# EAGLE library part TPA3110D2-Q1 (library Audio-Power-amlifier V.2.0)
15-W Filter-Free Stereo Class-D Audio Power Amplifier with SpeakerGuard
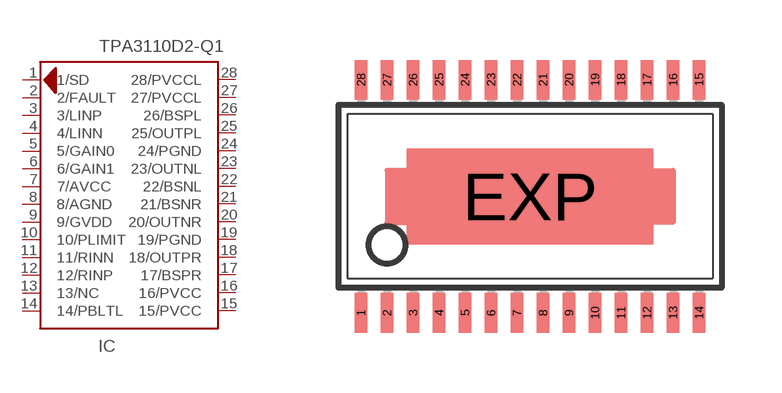
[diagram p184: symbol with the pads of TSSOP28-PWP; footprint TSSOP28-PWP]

Designator prefix IC

## TPA3110D2-Q1  [TSSOP28-PWP]
1  1/SD  out
2  2/FAULT  out
3  3/LINP  in
4  4/LINN  in
5  5/GAIN0
6  6/GAIN1
7  7/AVCC  pwr
8  8/AGND  pwr
9  9/GVDD  out
10  10/PLIMIT  in
11  11/RINN  in
12  12/RINP  in
13  13/NC  nc
14  14/PBLTL  in
15  15/PVCC  pwr
16  16/PVCC  pwr
17  17/BSPR  in
18  18/OUTPR  out
19  19/PGND  pwr
20  20/OUTNR  out
21  21/BSNR  in
22  22/BSNL  in
23  23/OUTNL  out
24  24/PGND  pwr
25  25/OUTPL  out
26  26/BSPL  in
27  27/PVCCL  pwr
28  28/PVCCL  pwr

## Footprint TSSOP28-PWP (pad centres in mm)
Power Thin Shrink Small Outline Plastic 28
smd 0.305 x 0.991: 1 -4.225,-2.918; 2 -3.575,-2.918; 3 -2.925,-2.918; 4 -2.275,-2.918; 5 -1.625,-2.918; 6 -0.975,-2.918; 7 -0.325,-2.918; 8 0.325,-2.918; 9 0.975,-2.918; 10 1.625,-2.918; 11 2.275,-2.918; 12 2.925,-2.918; 13 3.575,-2.918; 14 4.225,-2.918; 15 4.225,2.918; 16 3.575,2.918; 17 2.925,2.918; 18 2.275,2.918; 19 1.625,2.918; 20 0.975,2.918; 21 0.325,2.918; 22 -0.325,2.918; 23 -0.975,2.918; 24 -1.625,2.918; 25 -2.275,2.918; 26 -2.925,2.918; 27 -3.575,2.918; 28 -4.225,2.918
smd 6.17 x 2.4: EXP 0,0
